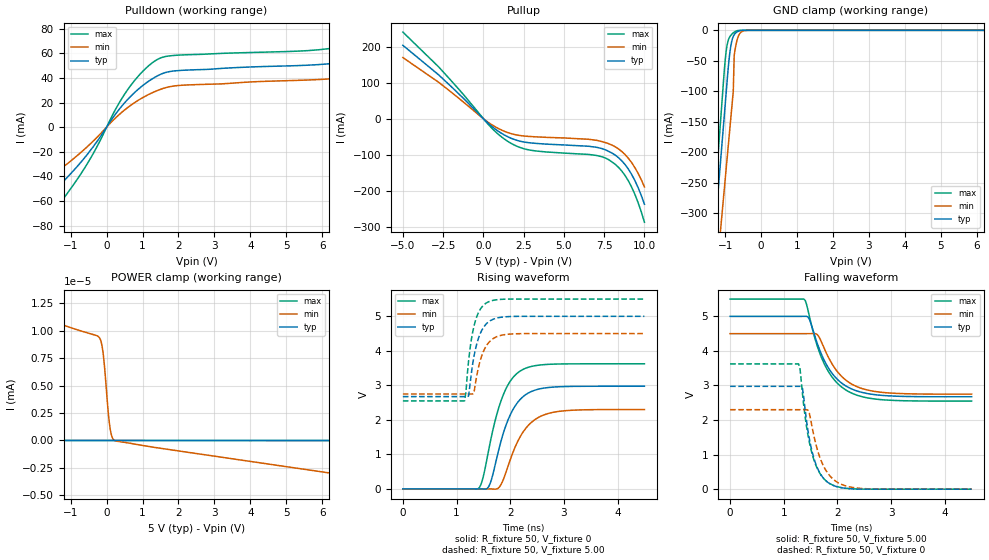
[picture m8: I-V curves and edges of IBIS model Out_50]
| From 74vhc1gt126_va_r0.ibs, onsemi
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|//////////////////////////////////////////////////////////////////////////////
|//////////////////////////////////////////////////////////////////////////////
[Model] Out_50
Model_type 3-state
Polarity Non-Inverting
Enable Active-High
Vmeas = 2.50
Vref = 5.0
Rref = 1k
Cref = 15pF
|  variable   typ   min   max
C_comp   3.8pF   3.8pF   3.8pF
|//////////////////////////////////////////////////////////////////////////////
[Temperature Range]   25   125   -55
|//////////////////////////////////////////////////////////////////////////////
[Voltage Range]   5.00V   4.50V   5.50V
|//////////////////////////////////////////////////////////////////////////////
[Pulldown Reference]   0V   0V   0V
|//////////////////////////////////////////////////////////////////////////////
[Pullup Reference]   5.00V   4.50V   5.50V
|//////////////////////////////////////////////////////////////////////////////
[GND Clamp Reference]   0V   0V   0V
|//////////////////////////////////////////////////////////////////////////////
[POWER Clamp Reference] 5.00V   4.50V   5.50V
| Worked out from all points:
|   slope of the pulldown table from 0 to 0.75 V, typ, clamps not added: 27.5 ohm
|   slope of the pullup table from 0 to 0.75 V, typ, clamps not added: 25.7 ohm
|   GND clamp passes 1 mA (typ) near -0.61 V on its own axis
|   POWER clamp passes 1 mA (typ) near -4.97 V on its own axis
|   falling waveform, R_fixture 50, V_fixture 5.00: 20-80 % time 466ps typ, 472ps min, 463ps max; typ from 5 V to 2.67 V
|   falling waveform, R_fixture 50, V_fixture 0: 20-80 % time 239ps typ, 298ps min, 250ps max; typ from 2.98 V to 0 V
|   rising waveform, R_fixture 50, V_fixture 0: 20-80 % time 378ps typ, 421ps min, 372ps max; typ from 0 V to 2.98 V
|   rising waveform, R_fixture 50, V_fixture 5.00: 20-80 % time 192ps typ, 200ps min, 168ps max; typ from 2.67 V to 5 V
|//////////////////////////////////////////////////////////////////////////////
[Pulldown]
|   Voltage   I(typ)   I(min)   I(max)
-5.5V     -219.5mA   -132.6mA   -252.3mA
-4.15V    -165.1mA   -88.85mA   -193.1mA
-2.3V     -89.02mA   -54.01mA   -112.7mA
-2.1V     -79.79mA   -50.49mA   -103.3mA
-1.7V     -60.95mA   -42.77mA   -82.41mA
575mV     22.13mA    15.63mA    29.94mA
1.55V     43.44mA    31.19mA    56.66mA
5.9V      50.77mA    38.63mA    62.78mA
7.4V      57.64mA    43.49mA    72.27mA
8.9V      79.63mA    59.3mA     101.4mA
10.1V     115.7mA    86.06mA    147.3mA
11V       156.8mA    117.4mA    198.5mA
|//////////////////////////////////////////////////////////////////////////////
[Pullup]
|   Voltage   I(typ)   I(min)   I(max)
-5V       203.6mA    169.6mA    240.2mA
-2.775V   121.5mA    100.9mA    143.6mA
250mV     -10.7mA    -8.446mA   -13.12mA
1.55V     -50.82mA   -38.98mA   -63.82mA
2.9V      -66.92mA   -49.36mA   -87.12mA
7.05V     -79.5mA    -60.15mA   -102.2mA
7.6V      -86.77mA   -66.62mA   -109.4mA
8.2V      -101.4mA   -78.27mA   -127.1mA
8.8V      -127.4mA   -99.62mA   -157.7mA
9.2V      -154.1mA   -121.5mA   -189.2mA
9.6V      -190.2mA   -150.9mA   -231.8mA
10V       -237.2mA   -189.1mA   -287.1mA
|//////////////////////////////////////////////////////////////////////////////
[GND Clamp]
|   Voltage   I(typ)   I(min)   I(max)
-5V       -3.004A    -2.815A    -3.24A
-1.4V     -409.9mA   -501.5mA   -365mA
-1.3V     -337.9mA   -437.2mA   -285.2mA
-1.225V   -283.8mA   -389mA     -225.3mA
-1.1V     -193.8mA   -308.7mA   -125.5mA
-975mV    -103.7mA   -228.4mA   -35.08mA
-850mV    -28.03mA   -148.1mA   -8.752mA
-775mV    -9.907mA   -99.86mA   -4.121mA
-750mV    -7.161mA   -41.5mA    -2.983mA
-675mV    -2.773mA   -17.18mA   -761.8uA
-375mV    -856.7nA   -68.58uA   -1.413nA
10V       16.23pA    3.107nA    972.2fA
|//////////////////////////////////////////////////////////////////////////////
[POWER Clamp]
|   Voltage   I(typ)   I(min)   I(max)
-5V       1.409mA    26.99nA    34.96mA
-4.85V    7.053uA    24.7nA     31.64mA
-4.775V   2.927nA    23.7nA     29.87mA
-4.025V   391.8pA    17.39nA    4.495mA
-3.8V     240pA      16.27nA    15.67uA
-3.725V   204.8pA    15.94nA    156.8pA
-2.825V   42.18pA    13.14nA    11.84pA
-225mV    5.599pA    9.452nA    479.1fA
-100mV    5.32pA     8.027nA    464.7fA
100mV     4.875pA    1.029nA    441.6fA
225mV     4.597pA    -5.923pA   427.2fA
10V       -17.17pA   -4.769nA   -700.2fA
|//////////////////////////////////////////////////////////////////////////////
|//////////////////////////////////////////////////////////////////////////////
[Ramp]
|  variable   typ   min   max
dV/dt_f   1.395E+00/4.500E-10  1.050E+00/4.750E-10  1.770E+00/4.750E-10
dV/dt_r   1.785E+00/3.750E-10  1.380E+00/4.250E-10  2.175E+00/3.750E-10
R_load = 50
|/////////////////////////////////////////////////////////////////////////////
[Falling Waveform]
R_fixture = 50
V_fixture = 5.00
V_fixture_min = 4.50
V_fixture_max = 5.50
C_fixture = 0p
|   time   V(typ)   V(min)   V(max)
0s        5V         4.5V       5.5V
1.375ns   5.001V     4.5V       5.5V
1.425ns   5.001V     4.5V       5.343V
1.475ns   4.921V     4.5V       5.016V
1.625ns   4.214V     4.472V     4.138V
1.775ns   3.661V     4V         3.561V
2ns       3.175V     3.398V     3.064V
2.275ns   2.893V     3.032V     2.773V
2.9ns     2.706V     2.792V     2.58V
4.5ns     2.675V     2.75V      2.55V
|//////////////////////////////////////////////////////////////////////////////
[Falling Waveform]
R_fixture = 50
V_fixture = 0
C_fixture = 0p
|   time   V(typ)   V(min)   V(max)
0s        2.975V     2.3V       3.625V
1.275ns   2.975V     2.3V       3.624V
1.3ns     2.975V     2.3V       3.522V
1.35ns    2.905V     2.3V       2.73V
1.45ns    1.698V     2.287V     1.569V
1.525ns   1.1V       1.82V      1.036V
1.675ns   460.6mV    907.4mV    450mV
1.875ns   141.5mV    356.1mV    146.3mV
2.45ns    1.172mV    20.8mV     1.891mV
4.5ns     0V         0V         0V
|//////////////////////////////////////////////////////////////////////////////
[Rising Waveform]
R_fixture = 50
V_fixture = 0
C_fixture = 0p
|   time   V(typ)   V(min)   V(max)
0s        0V         0V         0V
1.425ns   445.8uV    69.84uV    39.66mV
1.5ns     -2.61mV    73.52uV    367.8mV
1.625ns   153.4mV    1.202mV    1.332V
1.85ns    1.504V     194.7mV    2.643V
2.025ns   2.223V     950.9mV    3.175V
2.225ns   2.653V     1.613V     3.451V
2.45ns    2.856V     1.998V     3.567V
2.8ns     2.951V     2.22V      3.615V
4.5ns     2.975V     2.3V       3.625V
|//////////////////////////////////////////////////////////////////////////////
[Rising Waveform]
R_fixture = 50
V_fixture = 5.00
V_fixture_min = 4.50
V_fixture_max = 5.50
C_fixture = 0p
|   time   V(typ)   V(min)   V(max)
0s        2.675V     2.75V      2.55V
1.15ns    2.675V     2.75V      2.55V
1.175ns   2.675V     2.75V      2.803V
1.225ns   2.692V     2.75V      3.716V
1.275ns   3.34V      2.75V      4.317V
1.325ns   3.842V     2.788V     4.716V
1.45ns    4.529V     3.765V     5.223V
1.6ns     4.843V     4.241V     5.423V
2.025ns   4.995V     4.489V     5.5V
4.5ns     5V         4.5V       5.5V
